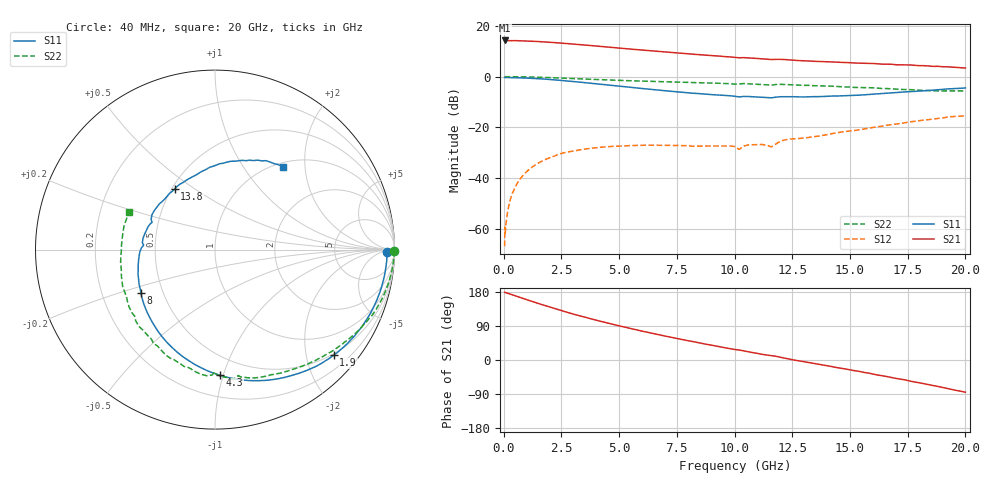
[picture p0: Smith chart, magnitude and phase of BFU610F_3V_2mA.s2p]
! Filename:  P:\Prog\Test\Noise\ATS_data\Testdata_Net\SplitFiles\BFU610_2W_A5_HighFreq_3V_2mA_D.s2p
! Date/Time: Wed 10/Aug/2011 16:57:15
! BFU610_2W_A5_HighFreq_3V_1mA_10mA_Bias2_R.s2p
! MDIF S-parameter v. bias file
! BFU610_2W_A5_HighFreq_3V_1mA_10mA
! Date/time Mon Aug 08 14:07:26 2011
! VAR V_out= 3.0000
! VAR I_out= 1.9900
! VAR V_in= 0.8655
! VAR I_in= 0.0148
! Device data file deembeded for feedlines and parallel
! Original file: \SplitFiles\BFU610_2W_A5_HighFreq_3V_2mA_R.s2p
! Feed-files: PR003V01_101208_Feed1.s2p, PR003V01_101208_Feed2.s2p
! Parallel-file: PR003V01_101208_Par.s2p
# MHz S MA R 50
!  Freq-MHz  S11-mag  S11-arg  S21-mag  S21-arg  S12-mag  S12-arg  S22-mag  S22-arg
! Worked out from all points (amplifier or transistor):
!   167 points, 40 MHz to 20 GHz, reference 50 ohm
!   highest |S21| = 14.3 dB at 40 MHz (marker M1)
!   |S21| within 3 dB of that: start of sweep to 4.997 GHz
!   unconditionally stable (mu >= 1): 6.807 GHz to 18.7 GHz
!   at 550 MHz: K = 0.01, MSG = 28.4 dB, |S12| = -42.7 dB
!   at 4.2 GHz: K = 0.52, MSG = 19.9 dB, |S12| = -27.9 dB
!   at 20 GHz: K = 0.89, MSG = 9.4 dB, |S12| = -15.5 dB
!   S11 on the Smith chart (normalised r, x): 40 MHz: 43, -15; 1.9 GHz: 0.47, -2.55; 4.3 GHz: 0.35, -0.97; 8 GHz: 0.38, -0.24; 13.8 GHz: 0.52, +0.42; 20 GHz: 1.07, +1.54
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40  0.9594 -0.8  5.17 178.7  0.0004524 87.1  0.9964 -0.4
50  0.9553 -0.9  5.143 178.9  0.001079 98.3  0.9967 -0.5
70  0.9592 -1.5  5.134 178.1  0.0008311 90.3  0.9972 -0.7
200  0.9585 -4.5  5.12 175.6  0.002573 90.9  0.9969 -2.1
480  0.9532 -10.8  5.107 169.8  0.006385 86.3  0.9947 -5.1
1150  0.9281 -25.6  5.015 156.1  0.01536 74.9  0.9815 -12.2
1900  0.8854 -41.6  4.791 141.4  0.02416 63.7  0.9598 -19.6
2700  0.824 -57.9  4.511 126.7  0.03228 52.4  0.9266 -27.0
3400  0.7703 -71.4  4.235 114.8  0.03654 44.7  0.9005 -33.0
4300  0.7002 -87.9  3.909 100.5  0.04079 36.0  0.8678 -40.0
5400  0.622 -107.0  3.529 84.4  0.04354 27.8  0.8326 -48.0
6800  0.5363 -130.2  3.106 65.7  0.0442 20.4  0.7938 -57.7
8000  0.4783 -149.7  2.802 50.7  0.0434 16.8  0.7633 -65.9
9400  0.4307 -171.6  2.528 34.4  0.04282 18.6  0.7368 -75.7
10200  0.3981 176.4  2.354 26.4  0.03671 20.7  0.7145 -79.5
11600  0.3819 156.5  2.175 11.4  0.04109 30.0  0.6807 -90.3
12000  0.4015 150.9  2.189 7.0  0.05369 37.6  0.7042 -93.7
13400  0.4029 129.1  2.01 -8.6  0.06513 31.1  0.6638 -107.1
13800  0.4049 123.8  1.973 -12.7  0.06888 31.4  0.6537 -110.6
16800  0.4795 86.7  1.754 -46.2  0.1133 18.4  0.5756 -146.2
18400  0.5339 69.0  1.623 -65.3  0.1422 5.2  0.5316 -171.6
20000  0.5976 50.7  1.476 -85.0  0.1686 -11.6  0.5216 156.6
